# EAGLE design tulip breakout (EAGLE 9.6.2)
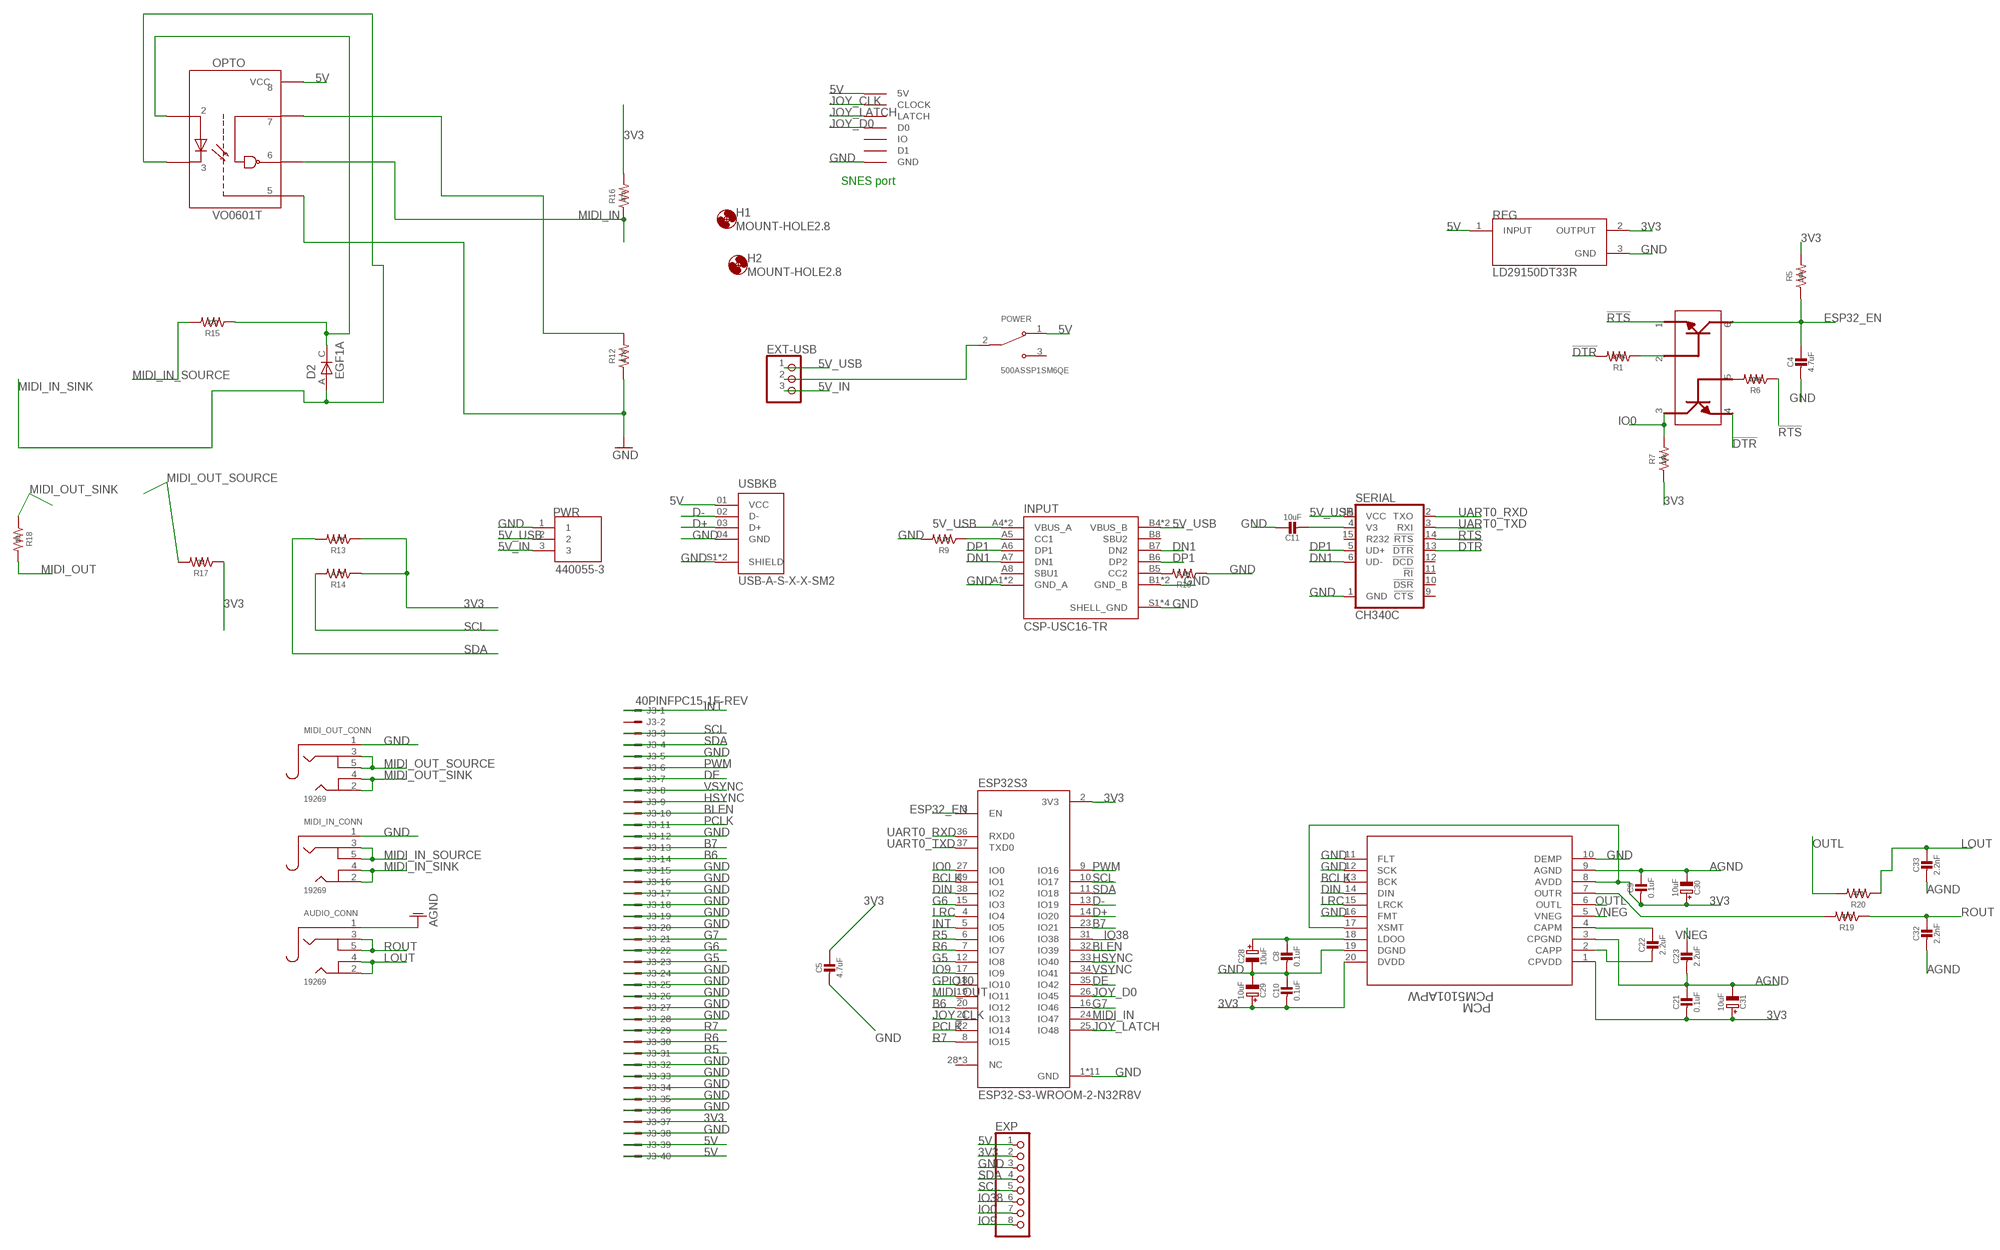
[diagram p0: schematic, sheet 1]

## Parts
AUDIO_CONN  19269  AUDIO_3.5MMJACK  [4UCONN_19269]
C4  4.7uF  CAP_CERAMIC0805-NOOUTLINE  [0805-NO]
C5  4.7uF  CAP_CERAMIC0805-NOOUTLINE  [0805-NO]
C8  0.1uF  CAP_CERAMIC0805-NOOUTLINE  [0805-NO]
C9  0.1uF  CAP_CERAMIC0805-NOOUTLINE  [0805-NO]
C10  0.1uF  CAP_CERAMIC0805-NOOUTLINE  [0805-NO]
C11  10uF  CAP_CERAMIC0805-NOOUTLINE  [0805-NO]
C21  0.1uF  CAP_CERAMIC0805-NOOUTLINE  [0805-NO]
C22  2.2uF  CAP_CERAMIC0805-NOOUTLINE  [0805-NO]
C23  2.2uF  CAP_CERAMIC0805-NOOUTLINE  [0805-NO]
C28  10uF  CAP_ELECTROLYTICPANASONIC_C  [PANASONIC_C]
C29  10uF  CAP_ELECTROLYTICPANASONIC_C  [PANASONIC_C]
C30  10uF  CAP_ELECTROLYTICPANASONIC_C  [PANASONIC_C]
C31  10uF  CAP_ELECTROLYTICPANASONIC_C  [PANASONIC_C]
C32  2.2nF  CAP_CERAMIC0805-NOOUTLINE  [0805-NO]
C33  2.2nF  CAP_CERAMIC0805-NOOUTLINE  [0805-NO]
D2  EGF1A  [DIOM449X264X300L114X135N]
ESP32S3  ESP32-S3-WROOM-2-N32R8V  [XCVR_ESP32-S3-WROOM-2-N32R8V]
EXP  PINHD-1X8BIG  [1X08-BIG]
EXT-USB  PINHD-1X3  [1X03]
H1  MOUNT-HOLE2.8  [2,8]
H2  MOUNT-HOLE2.8  [2,8]
INPUT  CSP-USC16-TR  [VALCON_CSP-USC16-TR]
J3  40PINFPC15-1F-REV  [XF2M-4015-1F-REVERSE]
MIDI_IN_CONN  19269  AUDIO_3.5MMJACK  [4UCONN_19269]
MIDI_OUT_CONN  19269  AUDIO_3.5MMJACK  [4UCONN_19269]
OPTO  VO0601T  [SOIC127P610X331-8N]
PCM  PCM5101APW  [PW20_TEX]
POWER  500ASSP1SM6QE  [SW_500ASSP1SM6QE]
PWR  440055-3  [TE_440055-3]
R1  100k  R-US_R0805  [R0805]
R5  10k  R-US_R0805  [R0805]
R6  100k  R-US_R0805  [R0805]
R7  10k  R-US_R0805  [R0805]
R9  5.1K  R-US_R0805  [R0805]
R10  5.1K  R-US_R0805  [R0805]
R12  4.7K  R-US_R0805  [R0805]
R13  4.7K  R-US_R0805  [R0805]
R14  4.7K  R-US_R0805  [R0805]
R15  220  R-US_R0805  [R0805]
R16  470  R-US_R0805  [R0805]
R17  33  R-US_R0805  [R0805]
R18  10  R-US_R0805  [R0805]
R19  470  R-US_R0805  [R0805]
R20  470  R-US_R0805  [R0805]
REG  LD29150DT33R  [DPAK456P972X240-3N]
RESET  MBT3904DW1T1G  [SOT236]
SERIAL  CH340C  [SO016]
SNES  SNESCONN  [SNESCONN]
USBKB  USB-A-S-X-X-SM2  [SAMTEC_USB-A-S-X-X-SM2]

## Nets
3V3: C5.1 C9.2 C10.2 C21.2 C29.+ C30.+ C31.+ ESP32S3.2(3V3) EXP.2 J3.37 PCM.1(CPVDD) PCM.8(AVDD) PCM.17(XSMT) PCM.20(DVDD) R5.2 R7.1 R13.1 R14.1 R16.2 R17.1 REG.2(OUTPUT)
5V: EXP.1 J3.39 J3.40 OPTO.8(VCC) POWER.1(NC) REG.1(INPUT) SNES.5V USBKB.01(VCC)
5V_IN: EXT-USB.3 PWR.3
5V_USB: EXT-USB.1 INPUT.A4(VBUS_A) INPUT.A9(VBUS_A) INPUT.B4(VBUS_B) INPUT.B9(VBUS_B) PWR.2 SERIAL.16(VCC)
!DTR: R1.2 RESET.4 SERIAL.13(!DTR)
!RTS: R6.1 RESET.1 SERIAL.14(!RTS)
AGND: AUDIO_CONN.1 C9.1 C21.1 C23.2 C30.- C31.- C32.2 C33.2 PCM.3(CPGND) PCM.9(AGND)
B6: ESP32S3.20(IO12) J3.14
B7: ESP32S3.23(IO21) J3.13
BCLK: ESP32S3.39(IO1) PCM.13(BCK)
BLEN: ESP32S3.32(IO39) J3.10
D+: ESP32S3.14(IO20) USBKB.03(D+)
D-: ESP32S3.13(IO19) USBKB.02(D-)
DE: ESP32S3.35(IO42) J3.7
DIN: ESP32S3.38(IO2) PCM.14(DIN)
DN1: INPUT.A7(DN1) INPUT.B7(DN2) SERIAL.6(UD-)
DP1: INPUT.A6(DP1) INPUT.B6(DP2) SERIAL.5(UD+)
ESP32_EN: C4.1 ESP32S3.3(EN) R5.1 RESET.6
EXT-USB: EXT-USB.2 POWER.2(COM)
G5: ESP32S3.12(IO8) J3.23
G6: ESP32S3.15(IO3) J3.22
G7: ESP32S3.16(IO46) J3.21
GND: C4.2 C5.2 C8.2 C10.1 C11.1 C28.- C29.- ESP32S3.1(GND) ESP32S3.40(GND) ESP32S3.41_1(GND) ESP32S3.41_2(GND) ESP32S3.41_3(GND) ESP32S3.41_4(GND) ESP32S3.41_5(GND) ESP32S3.41_6(GND) ESP32S3.41_7(GND) ESP32S3.41_8(GND) ESP32S3.41_9(GND) EXP.3 INPUT.A1(GND_A) INPUT.A12(GND_A) INPUT.B1(GND_B) INPUT.B12(GND_B) INPUT.S1(SHELL_GND) INPUT.S2(SHELL_GND) INPUT.S3(SHELL_GND) INPUT.S4(SHELL_GND) J3.5 J3.12 J3.15 J3.16 J3.17 J3.18 J3.19 J3.20 J3.24 J3.25 J3.26 J3.27 J3.28 J3.32 J3.33 J3.34 J3.35 J3.36 J3.38 MIDI_IN_CONN.1 MIDI_OUT_CONN.1 OPTO.5(GND) PCM.10(DEMP) PCM.11(FLT) PCM.12(SCK) PCM.16(FMT) PCM.19(DGND) PWR.1 R9.2 R10.1 R12.1 REG.3(GND) SERIAL.1(GND) SNES.GND USBKB.04(GND) USBKB.S1(SHIELD) USBKB.S2(SHIELD)
GPIO10: ESP32S3.18(IO10)
HSYNC: ESP32S3.33(IO40) J3.9
INT: ESP32S3.5(IO5) J3.1
IO0: ESP32S3.27(IO0) EXP.7 R7.2 RESET.3
IO9: ESP32S3.17(IO9) EXP.8
IO38: ESP32S3.31(IO38) EXP.6
JOY_CLK: ESP32S3.21(IO13) SNES.CLOCK
JOY_D0: ESP32S3.26(IO45) SNES.D0
JOY_LATCH: ESP32S3.25(IO48) SNES.LATCH
LOUT: AUDIO_CONN.2 AUDIO_CONN.4 C33.1 R20.1
LRC: ESP32S3.4(IO4) PCM.15(LRCK)
MIDI_IN: ESP32S3.24(IO47) OPTO.6(VO) R16.1
MIDI_IN_SINK: D2.A MIDI_IN_CONN.2 MIDI_IN_CONN.4 OPTO.3(C)
MIDI_IN_SOURCE: MIDI_IN_CONN.3 MIDI_IN_CONN.5 R15.2
MIDI_OUT: ESP32S3.19(IO11) R18.2
MIDI_OUT_SINK: MIDI_OUT_CONN.2 MIDI_OUT_CONN.4 R18.1
MIDI_OUT_SOURCE: MIDI_OUT_CONN.3 MIDI_OUT_CONN.5 R17.2
N$1: R1.1 RESET.2
N$2: R6.2 RESET.5
N$3: INPUT.B5(CC2) R10.2
N$7: C8.1 C28.+ PCM.18(LDOO)
N$8: PCM.7(OUTR) R19.2
N$16: C22.1 PCM.4(CAPM)
N$18: C22.2 PCM.2(CAPP)
N$30: D2.C OPTO.2(A) R15.1
N$32: OPTO.7(VE) R12.2
N$38: C11.2 SERIAL.4(V3)
N$42: INPUT.A5(CC1) R9.1
OUTL: PCM.6(OUTL) R20.2
PCLK: ESP32S3.22(IO14) J3.11
PWM: ESP32S3.9(IO16) J3.6
R5: ESP32S3.6(IO6) J3.31
R6: ESP32S3.7(IO7) J3.30
R7: ESP32S3.8(IO15) J3.29
ROUT: AUDIO_CONN.3 AUDIO_CONN.5 C32.1 R19.1
SCL: ESP32S3.10(IO17) EXP.5 J3.3 R14.2
SDA: ESP32S3.11(IO18) EXP.4 J3.4 R13.2
UART0_RXD: ESP32S3.36(RXD0) SERIAL.2(TXO)
UART0_TXD: ESP32S3.37(TXD0) SERIAL.3(RXI)
VNEG: C23.1 PCM.5(VNEG)
VSYNC: ESP32S3.34(IO41) J3.8
Unconnected: ESP32S3.28(NC) ESP32S3.29(NC) ESP32S3.30(NC) INPUT.A8(SBU1) INPUT.B8(SBU2) J3.2 POWER.3(NO) SERIAL.9(!CTS) SERIAL.10(!DSR) SERIAL.11(!RI) SERIAL.12(!DCD) SERIAL.15(R232) SNES.D1 SNES.IO

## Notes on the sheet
- SNES port

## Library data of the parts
AUDIO_CONN MIDI_IN_CONN MIDI_OUT_CONN = microbuilder:AUDIO_3.5MMJACK: 3.5MM Audio Jack These are normally connected as follows, from left-to right on the schematic symbol above: Tip: Left Audio Inner Ring: Right Audio Shell: Common/GND
C4 C5 C8-C11 C21-C23 C32 C33 = microbuilder:CAP_CERAMIC: Ceramic Capacitors
C28-C31 = microbuilder:CAP_ELECTROLYTIC: Electrolytic Capacitors
D2 = EGF1A:EGF1A: EGF1A Series 1 A 100 V 50 ns Surface Mount Fast Recovery Rectifier - DO-214AC Check availability; AVAILABILITY: In Stock; DESCRIPTION: Diode Standard 50 V 1A Surface Mount DO-214AC (SMA); MF: ON Semiconductor; MP: EGF1A; PACKAGE: SMA-2 ON Semiconductor; PRICE: None; PURCHASE-URL: https://pricing.snapeda.com/search/part/EGF1A/?ref=eda
ESP32S3 = ESP32-S3-WROOM-2-N32R8V:ESP32-S3-WROOM-2-N32R8V: Check availability; AVAILABILITY: In Stock; DESCRIPTION: Bluetooth, WiFi 802.11b/g/n, Bluetooth v5.0 Transceiver Module 2.4GHz PCB Trace Surface Mount; MF: Espressif Systems; MP: ESP32-S3-WROOM-2-N32R8V; PACKAGE: Package; PRICE: None; PURCHASE-URL: https://pricing.snapeda.com/search/part/ESP32-S3-WROOM-2-N32R8V/?ref=eda
EXP = adafruit:PINHD-1X8: PIN HEADER
EXT-USB = adafruit:PINHD-1X3: PIN HEADER
H1 H2 = holes:MOUNT-HOLE: MOUNTING HOLE with drill center marker
INPUT = CSP-USC16-TR:CSP-USC16-TR: CSP-USC16-TR Valcon USB Type C Surface Mount PCB Socket Check availability; AVAILABILITY: In Stock; DESCRIPTION: CSP-USC16-TR Valcon USB Type C Surface Mount PCB Socket; MF: Valcon; MP: CSP-USC16-TR; PACKAGE: None; PRICE: None; PURCHASE-URL: https://pricing.snapeda.com/search/part/CSP-USC16-TR/?ref=eda
J3 = adafruit:40PINFPC: OMRON FPC Connector Source : http://www.omron.com/ecb/products/pdf/fpc.pdf XF2M-4015-rev is good for connecting up 'PSP' SHARP LQ043 LCDs
OPTO = VO0601T:VO0601T: High Speed Optocoupler, 10 MBd, SOIC-8 Package; DESCRIPTION: Logic Output Optoisolator 10MBd Open Drain 4000Vrms 1 Channel 5kV/µs CMTI 8-SOIC; DIGI-KEY_PART_NUMBER: 751-1377-2-ND; MF: Vishay Semiconductors; MP: VO0601T; PACKAGE: None; PURCHASE-URL: https://pricing.snapeda.com/search/part/VO0601T/?ref=eda
PCM = pcm5101apw:PCM5101APW; COPYRIGHT: Copyright (C) 2022 Ultra Librarian. All rights reserved.; DIGI-KEY_PART_NUMBER_1: PCM5101APW-ND; MANUFACTURER_PART_NUMBER: PCM5101APW; MFR_NAME: Texas Instruments
POWER = 500ASSP1SM6QE:500ASSP1SM6QE; DESCRIPTION: Slide Switch SPDT Surface Mount, Right Angle; DIGI-KEY_PART_NUMBER: EG5810TR-ND; MF: E-Switch; MP: 500ASSP1SM6QE; PACKAGE: None; PURCHASE-URL: https://pricing.snapeda.com/search/part/500ASSP1SM6QE/?ref=eda
PWR = 440055-3:440055-3; COMMENT: 440055-3; DESCRIPTION: Connector Header Through Hole, Right Angle 3 position 0.079 (2.00mm); DIGI-KEY_PART_NUMBER: A100044-ND; EU_ROHS_COMPLIANCE: Compliant; MF: TE Connectivity; MP: 440055-3; PACKAGE: None; PURCHASE-URL: https://pricing.snapeda.com/search/part/440055-3/?ref=eda
R1 R5-R7 R9 R10 R12-R20 = adafruit:R-US_: RESISTOR, American symbol
REG = LD29150DT33R:LD29150DT33R: LD29150 Series 1.5 A 3.3 V Fixed Output SMT LDO Voltage Regulator - TO-252; DESCRIPTION: Linear Voltage Regulator IC Positive Fixed 1 Output 1.5A DPAK; DIGI-KEY_PART_NUMBER: 497-1496-2-ND; MF: STMicroelectronics; MP: LD29150DT33R; PACKAGE: TO-252 STMicroelectronics; PURCHASE-URL: https://pricing.snapeda.com/search/part/LD29150DT33R/?ref=eda
RESET = MBT3904DW1T1G:MBT3904DW1T1G: Check availability; AVAILABILITY: In Stock; DESCRIPTION: Bipolar (BJT) Transistor Array 2 NPN (Dual) 40V 200mA 300MHz 150mW Surface Mount SC-88/SC70-6/SOT-363; MF: ON Semiconductor; MP: MBT3904DW1T1G; PACKAGE: SC-88-6 ON Semiconductor; PRICE: None; PURCHASE-URL: https://pricing.snapeda.com/search/part/MBT3904DW1T1G/?ref=eda
SERIAL = SparkFun-IC-Comms:CH340C; PROD_ID: IC-14038
SNES = gamepad-conn:SNESCONN
USBKB = USB-A-S-X-X-SM2:USB-A-S-X-X-SM2: USB-A (USB TYPE-A) USB 2.0 Receptacle Connector 4 Position Surface Mount, Right Angle; Through Hole Check availability; AVAILABILITY: In Stock; DESCRIPTION: USB-A (USB TYPE-A) USB 2.0 Receptacle Connector 4 Position Surface Mount, Right Angle; MF: Samtec; MP: USB-A-S-F-W-SM2-TR; PACKAGE: None; PRICE: None; PURCHASE-URL: https://pricing.snapeda.com/search/part/USB-A-S-F-W-SM2-TR/?ref=eda

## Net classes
1 power: width 0.178 mm

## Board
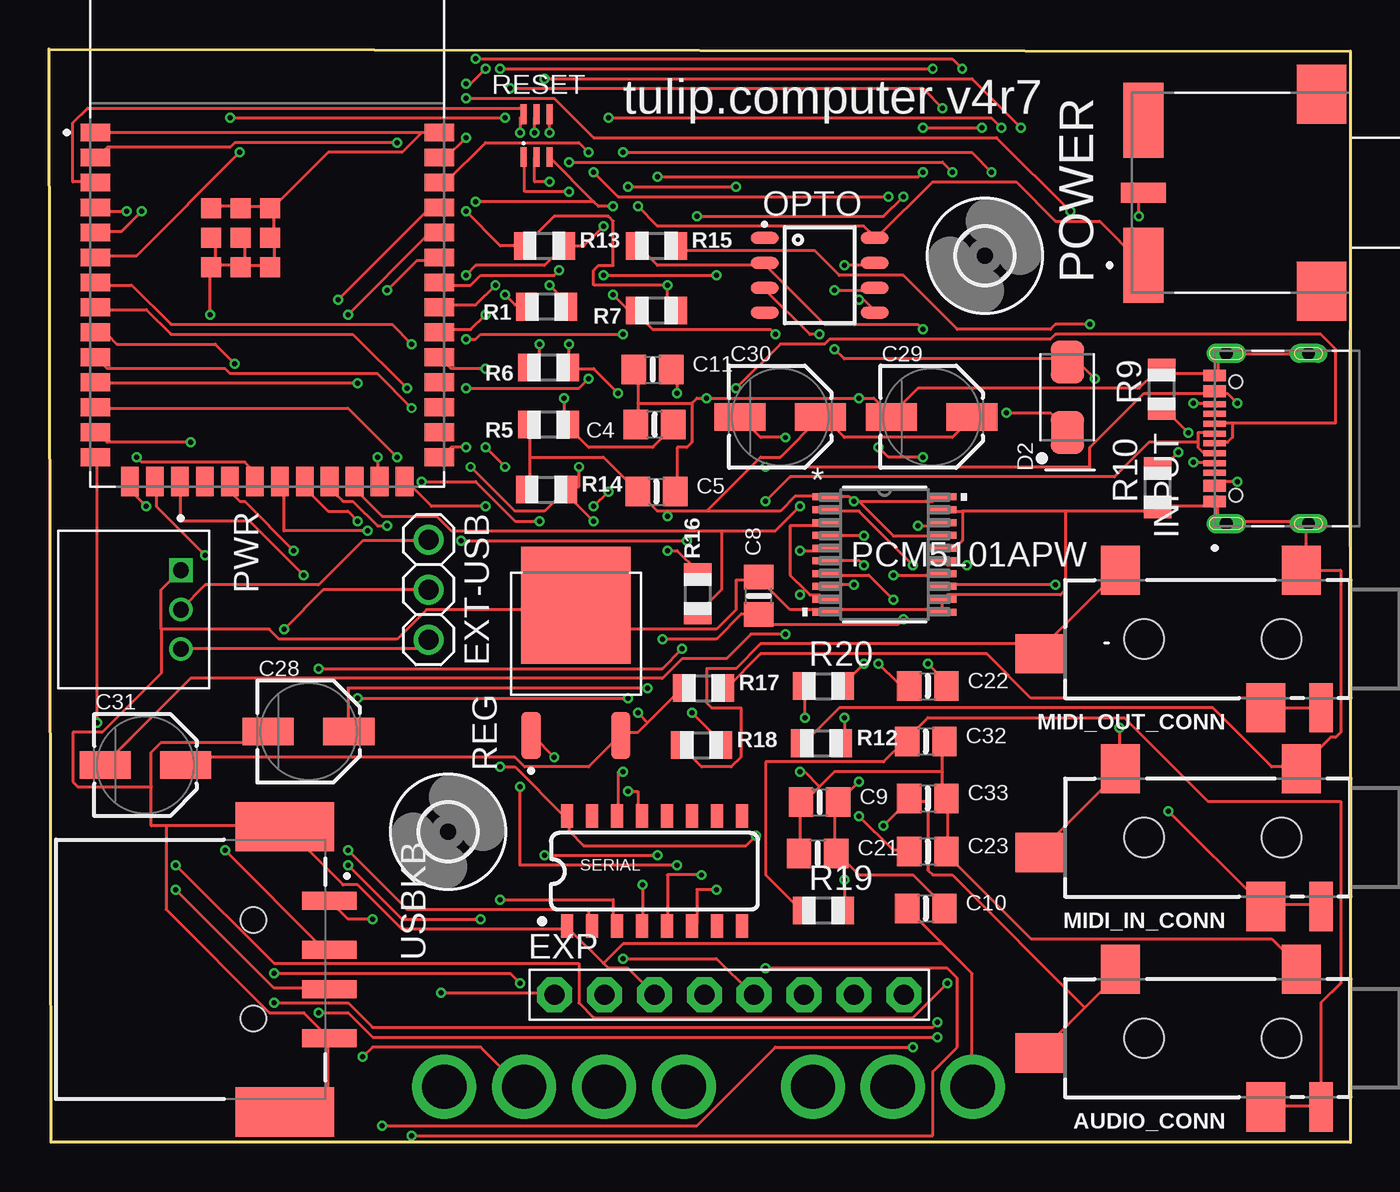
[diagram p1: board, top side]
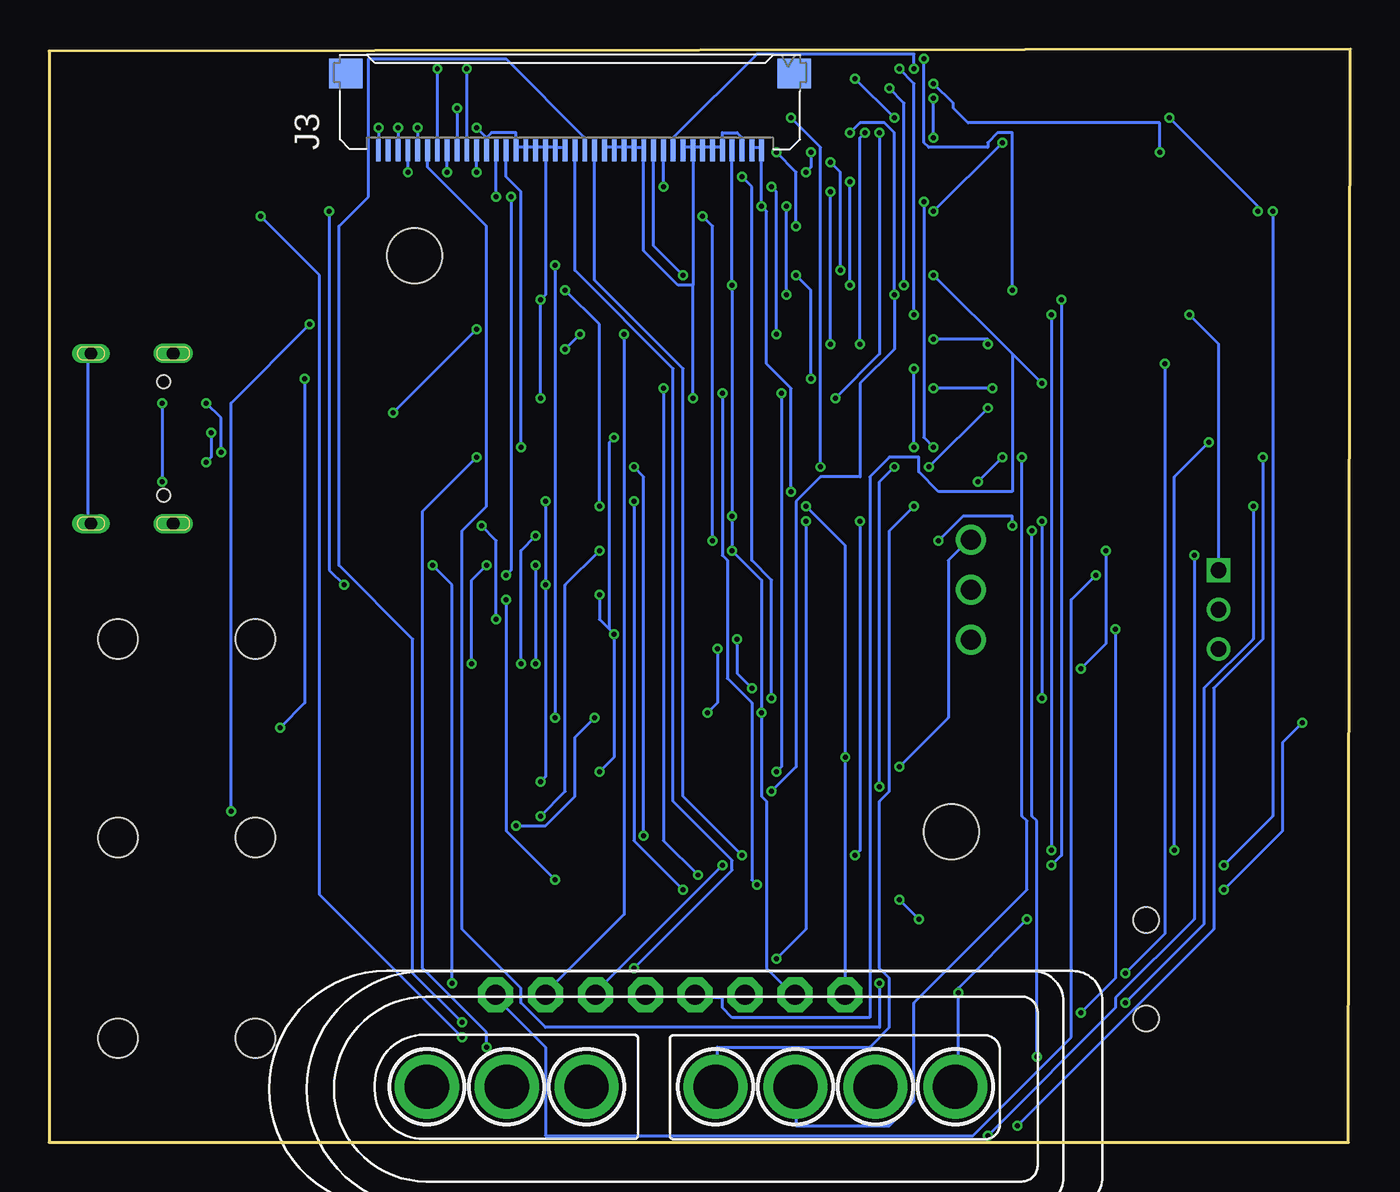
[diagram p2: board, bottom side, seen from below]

Size 66.2 x 55.6 mm. Coordinates in mm from the lower left corner, seen from the top.
Outline: 0.1,0 0,55.6 66.2,55.5 66.2,0 0.1,0
Copper layers (1*16): Top 0.035559375mm / dielectric 1.6mm / Bottom 0.035559375mm
Design rules "oshpark-2layer *": minimum track width 6mil, minimum drill 10mil, track to track 6mil, track to pad 6mil, pad to pad 6mil, via to via 6mil, smd to smd 6mil, copper to edge 0mil, drill to drill 6mil, minimum pad ring 5mil, minimum via ring 5mil, stop-mask expansion 2.5mil, vias tented up to drill 0mil, thermal gap 10mil

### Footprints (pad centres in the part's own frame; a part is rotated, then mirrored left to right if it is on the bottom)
4UCONN_19269 = smd 2 x 2.5: 1 2.5,-3.5; 2 11.7,-3.5; 3 4.3,3.5 | smd 2.5 x 2: 4 15.8,0.75 | smd 1.2 x 2.5: 5 1.5,3.5 | hole 2: 3.5,0; 10.5,0
0805-NO = smd 1.24 x 1.5: 1 -0.95,0; 2 0.95,0
PANASONIC_C = smd 2.6 x 1.4: + 2.05,0; - -2.05,0
DIOM449X264X300L114X135N = smd 2.17 x 1.69: A 1.795,0; C -1.795,0
XCVR_ESP32-S3-WROOM-2-N32R8V = smd 1.5 x 0.9: 1 -8.75,5.26; 2 -8.75,3.99; 3 -8.75,2.72; 4 -8.75,1.45; 5 -8.75,0.18; 6 -8.75,-1.09; 7 -8.75,-2.36; 8 -8.75,-3.63; 9 -8.75,-4.9; 10 -8.75,-6.17; 11 -8.75,-7.44; 12 -8.75,-8.71; 13 -8.75,-9.98; 14 -8.75,-11.25; 27 8.75,-11.25; 28 8.75,-9.98; 29 8.75,-8.71; 30 8.75,-7.44; 31 8.75,-6.17; 32 8.75,-4.9; 33 8.75,-3.63; 34 8.75,-2.36; 35 8.75,-1.09; 36 8.75,0.18; 37 8.75,1.45; 38 8.75,2.72; 39 8.75,3.99; 40 8.75,5.26 | smd 0.9 x 1.5: 15 -6.985,-12.5; 16 -5.715,-12.5; 17 -4.445,-12.5; 18 -3.175,-12.5; 19 -1.905,-12.5; 20 -0.635,-12.5; 21 0.635,-12.5; 22 1.905,-12.5; 23 3.175,-12.5; 24 4.445,-12.5; 25 5.715,-12.5; 26 6.985,-12.5 | smd 1 x 1: 41_1 -1.36,-0.09; 41_2 -2.86,-0.09; 41_3 0.14,-0.09; 41_4 -2.86,-1.59; 41_5 -1.36,-1.59; 41_6 0.14,-1.59; 41_7 -2.86,1.41; 41_8 -1.36,1.41; 41_9 0.14,1.41
1X08-BIG = drill 1.016 pad 1.778 octagon: 1 -8.89,0; 2 -6.35,0; 3 -3.81,0; 4 -1.27,0; 5 1.27,0; 6 3.81,0; 7 6.35,0; 8 8.89,0
1X03 = drill 1.016: 1 -2.54,0; 2 0,0; 3 2.54,0
2,8 = hole 2.8: 0,0
VALCON_CSP-USC16-TR = smd 0.3 x 1.14: A1 -3.35,0; A4 -2.55,0; A5 -1.25,0; A6 -0.25,0; A7 0.25,0; A8 1.25,0; A9 2.55,0; A12 3.35,0; B1 3.05,0; B4 2.25,0; B5 1.75,0; B6 0.75,0; B7 -0.75,0; B8 -1.75,0; B9 -2.25,0; B12 -3.05,0 | drill 0.65 pad 1 long: S1 -4.325,-0.59; S2 4.325,-0.59 | drill 0.65 pad 0.9 long: S3 -4.325,-4.77; S4 4.325,-4.77 | hole 0.65: -2.89,-1.07; 2.89,-1.07
XF2M-4015-1F-REVERSE = smd 1.1 x 0.25: 1 -2.54,9.75; 2 -2.54,9.25; 3 -2.54,8.75; 4 -2.54,8.25; 5 -2.54,7.75; 6 -2.54,7.25; 7 -2.54,6.75; 8 -2.54,6.25; 9 -2.54,5.75; 10 -2.54,5.25; 11 -2.54,4.75; 12 -2.54,4.25; 13 -2.54,3.75; 14 -2.54,3.25; 15 -2.54,2.75; 16 -2.54,2.25; 17 -2.54,1.75; 18 -2.54,1.25; 19 -2.54,0.75; 20 -2.54,0.25; 21 -2.54,-0.25; 22 -2.54,-0.75; 23 -2.54,-1.25; 24 -2.54,-1.75; 25 -2.54,-2.25; 26 -2.54,-2.75; 27 -2.54,-3.25; 28 -2.54,-3.75; 29 -2.54,-4.25; 30 -2.54,-4.75; 31 -2.54,-5.25; 32 -2.54,-5.75; 33 -2.54,-6.25; 34 -2.54,-6.75; 35 -2.54,-7.25; 36 -2.54,-7.75; 37 -2.54,-8.25; 38 -2.54,-8.75; 39 -2.54,-9.25; 40 -2.54,-9.75 | smd 1.5 x 1.7: M1 1.36,11.4; M2 1.36,-11.4
SOIC127P610X331-8N = smd 1.4 x 0.6: 1 -2.8,1.905; 2 -2.8,0.635; 3 -2.8,-0.635; 4 -2.8,-1.905; 5 2.8,-1.905; 6 2.8,-0.635; 7 2.8,0.635; 8 2.8,1.905
PW20_TEX = smd 1.473 x 0.356: 1 -2.921,2.925; 2 -2.921,2.275; 3 -2.921,1.625; 4 -2.921,0.975; 5 -2.921,0.325; 6 -2.921,-0.325; 7 -2.921,-0.975; 8 -2.921,-1.625; 9 -2.921,-2.275; 10 -2.921,-2.925; 11 2.921,-2.925; 12 2.921,-2.275; 13 2.921,-1.625; 14 2.921,-0.975; 15 2.921,-0.325; 16 2.921,0.325; 17 2.921,0.975; 18 2.921,1.625; 19 2.921,2.275; 20 2.921,2.925
SW_500ASSP1SM6QE = smd 3.81 x 2.03: 1 -3.685,4.535; 3 3.685,4.535 | smd 1.02 x 2.29: 2 0,4.535 | smd 3 x 2.5: S1 -5,-4.535; S2 5,-4.535
TE_440055-3 = drill 0.8 pad 1.15 square: 1 0,0 | drill 0.8 pad 1.15: 2 2.007,0; 3 4.013,0
R0805 = smd 1.1 x 1.4: 1 -1,0; 2 1,0
DPAK456P972X240-3N = smd 2.4 x 0.98: 1 -4.2,2.28; 2 -4.2,-2.28 | smd 5.96 x 5.57: 3 2.42,0
SOT236 = smd 0.3 x 1: 1 -0.66,-1.09; 2 0,-1.09; 3 0.66,-1.09; 4 0.66,1.09; 5 0,1.09; 6 -0.66,1.09
SO016 = smd 0.6 x 1.2: 1 -4.445,-2.8; 2 -3.175,-2.8; 3 -1.905,-2.8; 4 -0.635,-2.8; 5 0.635,-2.8; 6 1.905,-2.8; 7 3.175,-2.8; 8 4.445,-2.8; 9 4.445,2.8; 10 3.175,2.8; 11 1.905,2.8; 12 0.635,2.8; 13 -0.635,2.8; 14 -1.905,2.8; 15 -3.175,2.8; 16 -4.445,2.8
SNESCONN = drill 2.25 pad 3.25: 5V 0,4.064; CLOCK 4.064,4.064; D0 12.192,4.064; D1 18.756,4.064; GND 26.884,4.064; IO 22.82,4.064; LATCH 8.128,4.064
SAMTEC_USB-A-S-X-X-SM2 = smd 0.9 x 2.8: 01 -3.5,3.85; 02 -1,3.85; 03 1,3.85; 04 3.5,3.85 | smd 2.5 x 5: S1 -7.25,1.6; S2 7.25,1.6 | hole 1.3: -2.5,0; 2.5,0

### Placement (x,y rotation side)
AUDIO_CONN  66.2,5.3 180 top
C4  30.8,36.5 180 top
C5  30.9,33.1 0 top
C8  36.1,27.8 90 top
C9  39.2,17.3 0 top
C10  44.6,11.9 0 top
C11  30.7,39.3 0 top
C21  39.1,14.7 0 top
C22  44.7,23.2 0 top
C23  44.7,14.8 0 top
C28  13.2,20.9 0 top
C29  44.9,36.9 0 top
C30  37.2,36.9 0 top
C31  4.9,19.2 0 top
C32  44.6,20.4 0 top
C33  44.7,17.5 0 top
D2  51.8,37.9 90 top
ESP32S3  11.1,46.1 0 top
EXP  34.6,7.5 0 top
EXT-USB  19.3,28.1 270 top
H1  20.3,15.8 0 top
H2  47.6,45.1 0 top
INPUT  59.3,35.8 90 top
J3  39.7,53 90 bottom
MIDI_IN_CONN  66.2,15.5 180 top
MIDI_OUT_CONN  66.2,25.6 180 top
OPTO  39.2,44.1 0 top
PCM  42.5,29.9 0 top
POWER  60.2,48.3 90 top
PWR  6.7,29.1 270 top
R1  25.3,42.5 180 top
R5  25.4,36.5 180 top
R6  25.4,39.4 180 top
R7  30.9,42.3 180 top
R9  56.6,38.3 90 top
R10  56.4,33.3 90 top
R12  39.3,20.3 0 top
R13  25.2,45.6 0 top
R14  25.3,33.2 0 top
R15  30.9,45.6 0 top
R16  33,27.9 90 top
R17  33.3,23.1 0 top
R18  33.2,20.2 0 top
R19  39.4,11.8 0 top
R20  39.4,23.2 0 top
REG  26.8,24.9 90 top
RESET  24.8,51.2 0 top
SERIAL  30.8,13.8 0 top
SNES  20.1,6.9 180 bottom
USBKB  10.4,8.8 270 top

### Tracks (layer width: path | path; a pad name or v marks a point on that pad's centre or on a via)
3V3  (via drill 0.25)
  Top 0.152: C29.+ 46.95,36.85 45.95,35.85 40.45,35.85 39.45,36.85 C30.+ 37.2,34.85 36.2,34.85 33.45,32.1 | C10.2 45.45,12.1 43.95,13.6 41.2,13.6 40.2,14.6 C21.2 39.95,14.85 39.95,17.1 C9.2 v41.2,18.35 | 24.45,34.85 24.45,36.35 R5.2 | 24.45,34.85 24.45,33.35 R14.1 | 24.45,34.85 28.2,34.85 C5.1 30.95,32.1 31.45,32.1 | v40.95,28.35 39.7,28.35 PCM.8 | 41.2,32.6 42.95,30.85 45.2,30.85 PCM.17 | 41.2,32.6 44.95,32.6 45.2,32.85 PCM.20 | 41.2,32.6 v40.95,32.6 40.7,32.85 39.7,32.85 PCM.1 39.45,32.85 37.95,32.85 37.2,32.1 33.45,32.1 | 33.45,32.1 31.45,32.1 | 30.45,21.35 29.95,20.85 29.2,20.85 REG.2 28.95,20.6 27.45,19.1 24.2,19.1 23.7,19.6 7.2,19.6 6.95,19.35 C31.+ | 30.45,21.35 32.2,23.1 R17.1 | R7.1 31.7,42.35 31.45,42.35 v31.45,43.6 27.7,43.6 27.7,44.35 27.95,44.6 28.7,44.6 28.7,46.85 28.45,47.1 25.7,47.1 R13.1 22.95,45.6 v21.2,47.35 | v31.45,30.1 31.95,30.1 32.95,29.1 R16.2 | v17.7,50.85 9.45,50.85 9.2,50.6 2.95,50.6 2.45,50.1 ESP32S3.2 | v29.95,21.85 30.45,21.35 | v31.45,31.85 31.45,32.1
  Bottom 0.152: v40.95,32.6 v40.95,28.35 40.95,18.6 v41.2,18.35 | J3.37 v31.45,43.6 v31.45,31.85 v31.45,30.1 29.95,28.6 v29.95,21.85 29.95,17.6 29.7,17.35 29.7,8.85 28.45,7.6 EXP.2 | v21.2,47.35 v17.7,50.85
5V  (via drill 0.25)
  Top 0.152: v29.95,47.6 30.95,46.6 41.45,46.6 41.95,46.1 OPTO.8 42.2,46.1 44.95,48.85 49.2,48.85 51.2,46.85 53.45,46.85 55.45,44.85 POWER.1 | v25.7,19.6 24.7,20.6 REG.1 | USBKB.01 15.2,11.35 v16.45,11.35 | v19.95,7.6 25.7,7.6 EXP.1 | v27.7,32.35 v28.45,33.1
  Bottom 0.152: J3.39 30.45,50.6 29.95,50.6 J3.40 v29.95,47.6 29.7,47.35 29.7,39.6 28.45,38.35 v28.45,33.1 | EXP.1 25.7,7.6 v25.7,19.6 25.7,30.35 v27.7,32.35 | v16.45,11.35 19.95,7.85 v19.95,7.6 19.95,2.85 SNES.5V
5V_IN
  Top 0.152: PWR.3 18.95,25.1 19.2,25.35 EXT-USB.3
5V_USB  (via drill 0.25)
  Top 0.152: 59.45,33.6 59.45,33.35 INPUT.A4 | 59.45,38.1 59.45,38.35 INPUT.A9 | v60.45,33.6 59.45,33.6 | v60.45,37.6 59.95,38.1 59.45,38.1 | 59.45,33.6 INPUT.B9 | 59.45,38.1 INPUT.B4 59.2,38.1 55.7,38.1 52.95,35.35 52.95,34.35 v36.45,34.35 | v22.95,19.1 23.7,19.1 26.2,16.6 SERIAL.16 26.45,16.6 26.45,15.85 27.2,15.1 35.45,15.1 v35.95,15.6 | PWR.2 7.95,28.35 13.7,28.35 15.95,30.6 19.2,30.6 EXT-USB.1
  Bottom 0.152: v60.45,37.6 v60.45,33.6 | v22.95,19.1 20.45,21.6 20.45,29.6 19.45,30.6 EXT-USB.1 | v36.45,34.35 35.95,33.85 v35.95,15.6
!DTR  (via drill 0.25)
  Top 0.152: v25.45,51.35 25.45,52.1 RESET.4 | v23.2,43.1 23.7,42.6 24.2,42.6 R1.2 | v29.45,17.85 29.95,17.85 29.95,16.6 SERIAL.13
  Bottom 0.152: v25.45,51.35 24.95,51.85 23.7,51.85 23.2,51.35 v23.2,43.1 23.2,40.35 24.95,38.6 24.95,33.85 26.95,33.85 28.2,32.6 28.2,19.1 v29.45,17.85
!RTS  (via drill 0.25)
  Top 0.152: v26.45,48.35 24.2,48.35 24.2,50.1 RESET.1 | v26.45,40.6 26.45,39.6 R6.1 26.45,39.35 27.7,39.35 v28.95,38.1 | v29.2,18.85 28.95,18.85 28.95,16.6 SERIAL.14
  Bottom 0.152: v26.45,40.6 v26.45,48.35 | v29.2,18.85 28.95,19.1 v28.95,38.1
AGND  (via drill 0.25)
  Top 0.152: C21.1 38.2,14.85 38.2,17.1 C9.1 38.45,17.35 39.2,18.1 | 45.45,18.85 45.45,17.6 C33.2 45.7,17.35 45.7,14.85 C23.2 45.7,14.6 49.95,10.35 62.2,10.35 63.7,8.85 AUDIO_CONN.1 | 45.45,18.85 45.45,20.35 C32.2 | 39.2,18.1 39.95,18.85 45.45,18.85 | 38.45,28.1 37.7,28.85 37.7,31.35 39.45,31.35 PCM.3 | 38.45,28.1 38.7,27.85 39.2,27.85 39.45,27.6 PCM.9 | v37.45,25.85 35.7,25.85 34.45,24.6 32.2,24.6 31.2,23.6 7.2,23.6 2.95,19.35 C31.- | 38.45,28.1 v38.2,27.85 | C30.- 36.2,35.85 v37.45,35.85 | 39.2,18.1 38.45,18.85 v38.2,18.85
  Bottom 0.152: 37.7,26.1 38.2,26.6 v38.2,27.85 | 37.7,26.1 v37.45,25.85 37.45,19.6 v38.2,18.85 | v37.45,35.85 37.7,35.6 37.7,26.1
B6  (via drill 0.25)
  Top 0.152: v42.2,35.35 42.7,34.85 v44.45,34.85 | v43.95,4.85 36.95,4.85 32.95,0.85 v16.95,0.85 | v4.45,34.85 4.7,34.6 9.95,34.6 10.45,34.1 10.45,33.6 ESP32S3.20
  Bottom 0.152: J3.14 42.95,49.1 42.2,48.35 v42.2,35.35 | v44.45,34.85 47.2,32.1 47.2,8.85 43.95,5.6 v43.95,4.85 | v16.95,0.85 6.95,10.85 6.95,23.1 4.45,25.6 v4.45,34.85
B7  (via drill 0.25)
  Top 0.152: v43.45,48.1 42.45,47.1 v32.95,47.1 | v20.95,30.6 v32.45,30.6 | v17.2,31.35 16.7,31.35 15.45,32.6 14.95,32.6 14.45,33.1 14.45,33.6 ESP32S3.23
  Bottom 0.152: v43.45,48.1 J3.13 | v32.95,47.1 32.45,46.6 v32.45,30.6 | v20.95,30.6 19.7,31.85 17.2,31.85 v17.2,31.35
BCLK  (via drill 0.25)
  Top 0.152: v51.2,28.35 45.45,28.35 PCM.13 | v51.95,47.35 48.2,51.1 27.7,51.1 25.7,53.1 v21.2,53.1 | v21.2,51.1 20.2,50.1 19.95,50.1 ESP32S3.39
  Bottom 0.152: v51.2,28.35 51.95,29.1 v51.95,47.35 | v21.2,51.1 v21.2,53.1
BLEN  (via drill 0.25)
  Top 0.152: v22.95,54.6 v44.95,54.6 | v22.2,42.1 21.45,41.35 19.95,41.35 ESP32S3.32
  Bottom 0.152: v44.95,54.6 J3.10 | v22.95,54.6 22.2,53.85 v22.2,42.1
D+  (via drill 0.25)
  Top 0.152: v2.45,21.35 2.45,34.85 ESP32S3.14 | v6.45,12.85 11.45,7.85 14.2,7.85 USBKB.03
  Bottom 0.152: v2.45,21.35 3.45,20.35 3.45,15.85 v6.45,12.85
D-  (via drill 0.25)
  Top 0.152: v7.2,35.6 2.95,35.6 2.45,36.1 ESP32S3.13 | v8.95,14.85 13.95,9.85 14.2,9.85 USBKB.02
  Bottom 0.152: v7.2,35.6 8.95,33.85 v8.95,14.85
DE  (via drill 0.25)
  Top 0.152: v46.45,54.6 45.95,55.1 v21.7,55.1 | v17.2,43.35 18.7,44.85 19.7,44.85 ESP32S3.35
  Bottom 0.152: v46.45,54.6 J3.7 | v21.7,55.1 21.7,50.85 21.45,50.6 18.45,50.6 18.45,50.85 17.95,51.35 17.2,51.35 v17.2,43.35
DIN  (via drill 0.25)
  Top 0.152: v42.95,28.85 45.2,28.85 PCM.14 | v42.7,48.1 28.95,48.1 v27.7,49.35 | v27.45,50.35 26.95,50.85 22.2,50.85 20.2,48.85 19.95,48.85 ESP32S3.38
  Bottom 0.152: v42.95,28.85 42.7,29.1 v42.7,48.1 | v27.7,49.35 27.45,49.6 v27.45,50.35
DN1  (via drill 0.25)
  Top 0.152: 58.45,35.6 58.45,36.1 59.2,36.1 INPUT.A7 | 58.45,35.6 58.45,35.35 58.7,35.1 59.2,35.1 INPUT.B7 | v33.95,12.85 32.95,12.85 32.95,11.1 SERIAL.6 | v36.45,32.6 37.7,33.85 54.2,33.85 55.95,35.6 58.45,35.6
  Bottom 0.152: v33.95,12.85 36.45,15.35 v36.45,32.6
DP1  (via drill 0.25)
  Top 0.152: 60.2,36.6 60.2,35.85 59.95,35.6 59.45,35.6 INPUT.A6 | 60.2,36.6 59.45,36.6 INPUT.B6 | v33.2,13.6 31.45,13.6 31.45,11.1 SERIAL.5 | v34.95,38.35 37.2,40.6 39.45,40.6 39.7,40.85 50.95,40.85 51.2,41.1 64.7,41.1 65.45,40.35 65.45,36.6 60.2,36.6
  Bottom 0.152: v33.2,13.6 34.95,15.35 v34.95,38.35
ESP32_EN  (via drill 0.25)
  Top 0.152: C4.1 31.7,36.35 30.7,35.35 27.45,35.35 26.45,36.35 R5.1 26.2,36.6 v26.2,37.85 | ESP32S3.3 2.2,48.85 1.2,48.85 1.2,51.85 1.95,52.6 23.95,52.6 24.2,52.35 RESET.6 24.2,52.1 23.95,52.1 v23.95,51.35
  Bottom 0.152: v26.2,37.85 23.95,40.1 v23.95,51.35
EXT-USB  (via drill 0.25)
  Top 0.152: v55.45,47.1 55.45,48.1 POWER.2 | v45.2,5.35 16.45,5.35 15.2,6.6 v13.7,6.6 | v11.95,26.1 13.95,28.1 EXT-USB.2
  Bottom 0.152: v55.45,47.1 52.45,44.1 52.45,12.6 v45.2,5.35 | v13.7,6.6 11.95,8.35 v11.95,26.1
G5  (via drill 0.25)
  Top 0.152: v25.2,14.6 v30.95,14.6 | v24.95,31.6 23.7,31.6 21.7,33.6 v18.95,33.6 | v17.7,34.85 15.2,37.35 2.45,37.35 ESP32S3.12
  Bottom 0.152: J3.23 38.45,43.85 33.95,39.35 33.95,17.6 v30.95,14.6 | v25.2,14.6 24.95,14.85 v24.95,31.6 | v17.7,34.85 v18.95,33.6
G6  (via drill 0.25)
  Top 0.152: v45.2,6.1 44.95,5.85 16.45,5.85 15.2,7.1 v11.45,7.1 | v4.95,32.35 4.2,33.1 4.2,33.6 ESP32S3.15
  Bottom 0.152: J3.22 38.95,51.1 42.95,55.1 49.95,55.1 49.95,48.1 51.45,46.6 51.45,29.35 47.7,25.6 47.7,8.6 v45.2,6.1 | v11.45,7.1 7.45,11.1 7.45,23.1 4.95,25.6 v4.95,32.35
G7  (via drill 0.25)
  Top 0.152: v36.45,8.85 45.7,8.85 46.2,8.35 46.2,4.85 44.95,3.6 44.95,0.35 v18.45,0.35 | v7.95,29.85 5.45,32.35 5.45,33.6 ESP32S3.16
  Bottom 0.152: J3.21 39.45,44.35 34.45,39.35 34.45,17.35 31.45,14.35 31.45,13.85 v36.45,8.85 | v18.45,0.35 11.95,6.85 11.95,7.35 7.95,11.35 v7.95,29.85
GND  (via drill 0.25)
  Top 0.152: USBKB.S2 12.2,1.6 14.2,1.6 14.2,5.1 USBKB.04 12.95,6.6 11.2,6.6 5.95,11.85 5.95,16.1 | 5.2,18.1 5.2,16.1 5.95,16.1 | 5.2,18.1 5.2,19.85 5.7,20.35 10.45,20.35 10.95,20.85 C28.- | 5.95,16.1 11.95,16.1 USBKB.S1 14.95,13.1 15.7,13.1 17.95,10.85 26.2,10.85 SERIAL.1 26.45,10.85 28.2,9.1 | 28.2,9.1 28.45,8.85 29.45,8.85 30.7,7.6 EXP.3 | 45.45,10.1 46.95,8.6 46.95,2.85 SNES.GND | 45.45,10.1 C10.1 | 28.2,9.1 29.2,10.1 45.45,10.1 | ESP32S3.41_7 8.45,47.6 9.7,47.6 ESP32S3.41_8 9.95,47.6 11.2,47.6 ESP32S3.41_9 | 8.45,44.6 8.45,45.85 ESP32S3.41_2 | 9.95,44.6 9.95,45.85 ESP32S3.41_1 | 8.45,44.6 9.7,44.6 ESP32S3.41_5 9.95,44.6 | 8.45,44.6 ESP32S3.41_4 8.2,44.35 v8.2,42.1 | 9.95,44.6 11.2,44.6 ESP32S3.41_6 11.45,44.6 11.45,45.85 ESP32S3.41_3 11.45,46.1 11.45,47.35 ESP32S3.41_9 | 18.95,51.35 19.7,51.35 ESP32S3.40 | 18.95,51.35 2.45,51.35 ESP32S3.1 | 18.95,51.35 17.95,50.35 14.2,50.35 11.45,47.6 ESP32S3.41_9 | PWR.1 5.7,28.1 5.7,26.1 | 5.7,26.1 11.2,26.1 11.7,25.6 17.7,25.6 19.2,27.1 26.7,27.1 REG.3 26.95,27.1 27.95,26.1 33.95,26.1 34.95,27.1 34.95,28.6 35.95,28.6 C8.2 36.2,28.6 37.7,27.1 39.45,27.1 PCM.10 39.7,27.1 45.2,27.1 PCM.11 45.45,27.1 45.45,27.6 | v44.45,51.6 v47.45,51.6 | v41.2,42.85 41.45,42.85 41.95,42.35 OPTO.5 | 29.95,37.6 29.95,39.1 C11.1 | 29.95,37.6 29.95,36.6 C4.2 | 32.7,37.6 32.7,35.6 32.45,35.35 31.95,35.35 31.95,33.1 C5.2 | 29.95,37.6 32.7,37.6 | 32.7,37.6 32.95,37.85 v33.45,37.85 v41.2,37.85 41.95,37.85 42.7,37.1 C29.- 42.95,37.1 44.2,38.35 55.45,38.35 56.2,39.1 56.45,39.1 R9.2 56.7,39.1 59.2,39.1 INPUT.A12 59.45,39.1 | 63.7,19.1 62.2,19.1 59.2,22.1 40.2,22.1 38.45,20.35 R12.1
  Top 0.152: 59.45,39.1 59.45,38.85 INPUT.B1 | 59.45,39.1 59.45,40.1 59.7,40.1 INPUT.S2 59.95,40.1 63.95,40.1 INPUT.S4 | 63.95,29.1 63.95,31.35 INPUT.S3 63.95,31.6 59.95,31.6 INPUT.S1 59.7,31.6 59.45,31.6 59.45,32.35 | 46.45,32.1 46.45,30.6 46.2,30.35 45.45,30.35 PCM.16 | 46.45,32.1 45.45,32.1 PCM.19 | 59.45,32.35 59.45,32.85 INPUT.B12 | 59.45,32.35 INPUT.A1 59.2,32.35 56.45,32.35 R10.1 56.2,32.1 51.7,32.1 | 51.7,32.1 46.45,32.1 | 45.45,27.6 45.7,27.85 51.45,27.85 51.7,28.1 51.7,32.1 | 45.45,27.6 PCM.12 | 63.7,19.1 65.2,20.6 65.45,20.6 65.7,20.85 65.7,29.1 63.95,29.1 | 63.7,19.1 MIDI_IN_CONN.1 | 63.95,29.1 MIDI_OUT_CONN.1 | 5.2,18.1 1.45,18.1 1.2,18.35 1.2,20.85 2.7,20.85 5.7,23.85 5.7,26.1
  Bottom 0.152: v8.2,42.1 6.7,40.6 PWR.1 | 40.45,50.6 39.95,50.6 J3.20 | 40.45,50.6 40.95,50.6 | 40.45,50.6 J3.19 | 40.95,50.6 41.45,50.6 | 40.95,50.6 J3.18 40.95,43.1 v41.2,42.85 v41.2,37.85 | 41.45,50.6 41.95,50.6 | 41.45,50.6 J3.17 | 41.95,50.6 42.45,50.6 | 41.95,50.6 J3.16 | 43.95,51.1 J3.12 | 43.95,51.1 43.7,51.35 42.45,51.35 42.45,50.6 | 42.45,50.6 J3.15 | v47.45,51.6 J3.5 | 43.95,51.1 v44.45,51.6 | 36.45,50.6 35.95,50.6 J3.28 35.95,45.35 34.2,43.6 33.45,43.6 | 36.45,50.6 36.95,50.6 | 36.45,50.6 J3.27 | 36.95,50.6 37.45,50.6 | 36.95,50.6 J3.26 | 37.45,50.6 37.95,50.6 J3.24 | 37.45,50.6 J3.25 | J3.38 30.95,51.1 31.2,51.35 31.95,51.35 31.95,50.6 | 31.95,50.6 32.45,50.6 | 31.95,50.6 J3.36 | 32.45,50.6 32.95,50.6 | 32.45,50.6 J3.35 | 32.95,50.6 33.45,50.6 | 32.95,50.6 J3.34 | 33.45,50.6 33.95,50.6 J3.32 | 33.45,50.6 J3.33 33.45,43.6 | v33.45,37.85 33.45,43.6 | INPUT.S4 64.2,40.1 64.2,31.6 INPUT.S3
HSYNC  (via drill 0.25)
  Top 0.152: v45.45,52.6 44.45,53.6 v23.45,53.6 | v22.7,43.6 21.7,42.6 19.95,42.6 ESP32S3.33
  Bottom 0.152: v45.45,52.6 J3.9 | v23.45,53.6 22.7,52.85 v22.7,43.6
INT  (via drill 0.25)
  Top 0.152: v49.45,51.6 46.95,54.1 v25.2,54.1 | v9.2,52.1 v23.2,52.1 | v4.7,47.35 3.7,46.35 2.45,46.35 ESP32S3.5
  Bottom 0.152: v49.45,51.6 J3.1 | v23.2,52.1 v25.2,54.1 | v9.2,52.1 4.7,47.6 v4.7,47.35
IO0  (via drill 0.25)
  Top 0.152: 27.7,47.85 27.95,47.6 v28.7,47.6 | 27.7,47.85 RESET.3 | v28.7,43.1 29.45,42.35 29.7,42.35 R7.2 29.95,42.1 30.7,41.35 36.7,41.35 v36.95,41.1 | v21.2,35.35 20.45,35.35 19.95,34.85 ESP32S3.27 | 27.7,47.85 v21.7,47.85
  Bottom 0.152: v28.7,43.1 v28.7,47.6 | v21.2,35.35 21.7,35.85 v21.7,47.85 | v36.95,41.1 36.95,11.6 40.95,7.6 EXP.7
IO9  (via drill 0.25)
  Top 0.152: v12.95,28.85 10.2,31.6 6.7,31.6 6.7,33.6 ESP32S3.17
  Bottom 0.152: v12.95,28.85 14.2,27.6 14.2,5.35 19.2,0.35 40.95,0.35 40.95,4.85 43.45,7.35 EXP.8
IO38  (via drill 0.25)
  Top 0.152: v22.2,39.35 20.45,39.35 19.95,39.85 ESP32S3.31 | v23.2,34.35 v22.2,35.35 | v23.95,18.1 23.95,14.1 v31.95,14.1
  Bottom 0.152: v22.2,35.35 v22.2,39.35 | v23.2,34.35 23.95,33.6 v23.95,18.1 | v31.95,14.1 38.2,7.85 38.2,7.6 EXP.6
JOY_CLK  (via drill 0.25)
  Top 0.152: v16.2,31.1 11.95,31.1 11.95,33.6 ESP32S3.21 | v15.95,4.35 16.45,4.85 21.95,4.85 23.95,2.85 SNES.CLOCK
  Bottom 0.152: v16.2,31.1 16.2,16.6 15.95,16.35 v15.95,4.35
JOY_D0  (via drill 0.25)
  Top 0.152: v22.2,32.35 19.45,32.35 18.2,33.6 ESP32S3.26
  Bottom 0.152: v22.2,32.35 23.45,31.1 23.45,17.85 23.95,17.35 23.95,8.85 23.45,8.35 23.45,5.85 24.45,4.85 32.2,4.85 32.2,2.85 SNES.D0
JOY_LATCH  (via drill 0.25)
  Top 0.152: v16.7,34.85 16.7,33.6 ESP32S3.25
  Bottom 0.152: v16.7,34.85 16.7,16.6 16.45,16.35 16.45,12.85 22.2,7.1 22.2,2.1 23.45,0.85 28.2,0.85 28.2,2.6 SNES.LATCH
LOUT  (via drill 0.25)
  Top 0.152: 52.7,6.85 54.45,8.6 AUDIO_CONN.2 | 52.7,6.85 AUDIO_CONN.4 | v38.45,21.6 38.45,23.1 R20.1 | v42.45,16.1 43.7,17.35 C33.1 43.95,17.35 44.7,17.35 44.7,13.85 44.95,13.6 45.95,13.6 52.7,6.85
  Bottom 0.152: v38.45,21.6 39.45,20.6 39.45,17.6 40.95,16.1 v42.45,16.1
LRC  (via drill 0.25)
  Top 0.152: v46.7,29.35 45.7,29.35 45.45,29.6 PCM.15 | v45.7,8.1 43.95,6.35 27.7,6.35 26.95,7.1 26.95,9.1 11.45,9.1 v6.45,14.1 | v3.95,47.35 2.45,47.35 ESP32S3.4
  Bottom 0.152: v46.7,29.35 45.7,28.35 v45.7,8.1 | v6.45,14.1 3.95,16.6 v3.95,47.35
MIDI_IN  (via drill 0.25)
  Top 0.152: R16.1 34.2,28.1 34.2,31.1 | 34.2,31.1 20.45,31.1 19.7,31.85 16.95,31.85 15.7,33.1 15.7,33.6 ESP32S3.24 | v39.95,43.35 41.95,43.35 OPTO.6 | v38.2,32.35 36.95,31.1 34.2,31.1
  Bottom 0.152: v39.95,43.35 38.2,41.6 v38.2,32.35
MIDI_IN_SINK  (via drill 0.25)
  Top 0.152: MIDI_IN_CONN.4 50.45,14.85 54.45,18.85 MIDI_IN_CONN.2 54.45,19.1 v54.45,21.1 | v39.2,41.1 38.7,41.1 36.45,43.35 OPTO.3 | v39.95,40.35 40.45,39.85 51.7,39.85 D2.A 51.95,39.6 52.45,39.6 v53.2,38.85
  Bottom 0.152: v39.95,40.35 v39.2,41.1 | v54.45,21.1 53.2,22.35 v53.2,38.85
MIDI_IN_SOURCE  (via drill 0.25)
  Top 0.152: v52.95,41.6 51.2,41.6 50.95,41.35 46.2,41.35 43.45,44.1 40.2,44.1 38.95,45.35 32.2,45.35 31.95,45.6 R15.2 | v56.95,16.85 61.7,12.1 MIDI_IN_CONN.3 61.95,12.1 64.7,12.1 MIDI_IN_CONN.5
  Bottom 0.152: v52.95,41.6 56.95,37.6 v56.95,16.85
MIDI_OUT  (via drill 0.25)
  Top 0.152: v32.7,21.85 34.2,20.35 R18.2 | v32.2,25.1 31.2,24.1 v13.7,24.1 | v12.45,30.1 9.95,32.6 9.7,32.6 9.2,33.1 ESP32S3.19
  Bottom 0.152: v32.7,21.85 32.2,22.35 v32.2,25.1 | v13.7,24.1 12.45,25.35 v12.45,30.1
MIDI_OUT_SINK
  Top 0.152: 50.2,24.85 49.7,25.35 36.2,25.35 34.95,24.1 33.45,24.1 33.45,22.35 33.7,22.1 35.2,22.1 35.2,19.6 34.7,19.1 33.2,19.1 32.2,20.1 R18.1 | 50.2,24.85 54.45,29.1 MIDI_OUT_CONN.2 | 50.2,24.85 MIDI_OUT_CONN.4
MIDI_OUT_SOURCE
  Top 0.152: R17.2 34.45,23.1 36.2,24.85 47.7,24.85 49.95,22.6 61.2,22.6 61.7,22.1 MIDI_OUT_CONN.3 MIDI_OUT_CONN.5
N$1  (via drill 0.25)
  Top 0.152: v25.45,48.85 24.7,48.85 24.7,50.1 RESET.2 | v25.45,43.6 26.45,42.6 R1.1
  Bottom 0.152: v25.45,43.6 v25.45,48.85
N$2  (via drill 0.25)
  Top 0.152: v24.7,51.35 24.7,52.1 RESET.5 | v24.95,40.6 24.95,39.6 24.45,39.6 R6.2
  Bottom 0.152: v24.7,51.35 24.95,51.1 v24.95,40.6
N$3  (via drill 0.25)
  Top 0.152: v58.2,37.6 59.2,37.6 INPUT.B5 | v57.45,35.1 56.7,34.35 56.45,34.35 R10.2
  Bottom 0.152: v58.2,37.6 57.45,36.85 v57.45,35.1
N$7  (via drill 0.25)
  Top 0.152: v44.2,31.35 45.2,31.35 PCM.18 | v43.45,26.6 43.2,26.35 36.7,26.35 36.2,26.85 C8.1 35.2,26.85 33.95,25.6 v31.2,25.6 | v30.45,23.1 15.2,23.1 15.2,21.1 C28.+
  Bottom 0.152: v44.2,31.35 43.45,30.6 v43.45,26.6 | v30.45,23.1 31.2,23.85 v31.2,25.6
N$8  (via drill 0.25)
  Top 0.152: v40.45,13.35 40.45,11.85 R19.2 | v42.95,27.6 41.7,28.85 39.7,28.85 PCM.7
  Bottom 0.152: v40.45,13.35 42.95,15.85 v42.95,27.6
N$16  (via drill 0.25)
  Top 0.152: v41.45,30.85 39.7,30.85 PCM.4 | v42.2,24.35 43.2,23.35 43.7,23.35 C22.1
  Bottom 0.152: v41.45,30.85 42.2,30.1 v42.2,24.35
N$18  (via drill 0.25)
  Top 0.152: v43.95,29.35 41.2,32.1 39.7,32.1 PCM.2 | v44.7,24.35 45.7,23.35 C22.2
  Bottom 0.152: v43.95,29.35 44.7,28.6 v44.7,24.35
N$30  (via drill 0.25)
  Top 0.152: R15.1 29.95,45.6 30.95,44.6 36.2,44.6 OPTO.2 36.45,44.6 39.45,41.6 44.2,41.6 v44.45,41.35 | v48.7,37.1 50.95,37.1 51.7,36.35 D2.C
  Bottom 0.152: v44.45,41.35 v48.7,37.1
N$32  (via drill 0.25)
  Top 0.152: v40.45,21.6 40.45,20.35 R12.2 | v40.45,44.6 41.95,44.6 OPTO.7
  Bottom 0.152: v40.45,44.6 v40.45,21.6
N$38  (via drill 0.25)
  Top 0.152: v30.2,13.1 30.2,11.1 SERIAL.4 | v31.95,38.1 31.95,39.1 31.7,39.1 C11.2
  Bottom 0.152: v30.2,13.1 30.45,13.35 30.45,22.35 31.7,23.6 31.7,29.6 31.95,29.85 v31.95,38.1
N$42  (via drill 0.25)
  Top 0.152: v58.2,34.6 59.2,34.6 INPUT.A5 | v57.95,36.1 56.95,37.1 56.7,37.1 R9.1
  Bottom 0.152: v58.2,34.6 57.95,34.85 v57.95,36.1
OUTL  (via drill 0.25)
  Top 0.152: v41.45,24.35 40.45,23.35 R20.2 | v41.45,29.35 41.2,29.6 39.7,29.6 PCM.6
  Bottom 0.152: v41.45,29.35 v41.45,24.35
PCLK  (via drill 0.25)
  Top 0.152: v44.45,49.35 44.2,49.1 v30.95,49.1 | v15.7,22.6 v29.45,22.6 | v15.7,31.6 15.2,32.1 14.2,32.1 13.2,33.1 13.2,33.6 ESP32S3.22
  Bottom 0.152: v44.45,49.35 J3.11 | v30.95,49.1 30.45,48.6 30.45,29.6 29.45,28.6 v29.45,22.6 | v15.7,31.6 v15.7,22.6
PWM  (via drill 0.25)
  Top 0.152: v23.95,8.1 23.45,8.6 v11.45,8.6 | v9.45,39.6 8.45,40.6 3.45,40.6 2.95,41.1 2.45,41.1 ESP32S3.9
  Bottom 0.152: J3.6 46.95,49.6 43.95,46.6 43.95,32.35 45.2,31.1 45.2,10.85 42.2,7.85 42.2,7.1 40.95,5.85 23.95,5.85 v23.95,8.1 | v11.45,8.6 9.45,10.6 v9.45,39.6
R5  (via drill 0.25)
  Top 0.152: v22.2,54.6 21.45,53.85 v21.2,53.85 | v9.7,50.35 4.45,45.1 2.45,45.1 ESP32S3.6
  Bottom 0.152: J3.31 34.45,51.1 30.2,55.35 22.2,55.35 v22.2,54.6 | v21.2,53.85 20.2,52.85 20.2,52.6 19.45,51.85 9.7,51.85 v9.7,50.35
R6  (via drill 0.25)
  Top 0.152: v29.45,48.6 v34.95,48.6 | v29.2,41.1 21.95,41.1 21.7,40.85 v21.2,40.85 | v18.45,40.6 17.45,41.6 6.2,41.6 4.2,43.6 2.45,43.6 ESP32S3.7
  Bottom 0.152: v34.95,48.6 J3.30 | v29.45,48.6 29.2,48.35 v29.2,41.1 | v21.2,40.85 18.45,40.85 v18.45,40.6
R7  (via drill 0.25)
  Top 0.152: v28.2,44.1 v33.95,44.1 | v27.45,38.85 26.95,38.35 v21.2,38.35 | v18.2,38.35 15.45,41.1 6.2,41.1 4.95,42.35 2.45,42.35 ESP32S3.8
  Bottom 0.152: J3.29 35.45,45.6 v33.95,44.1 | v28.2,44.1 27.45,43.35 v27.45,38.85 | v18.2,38.35 v21.2,38.35
ROUT
  Top 0.152: 64.7,1.85 61.95,1.85 AUDIO_CONN.3 | R19.1 38.2,11.85 36.45,13.6 36.45,19.35 42.45,19.35 43.45,20.35 C32.1 43.7,20.6 44.7,21.6 54.7,21.6 58.95,17.35 65.7,17.35 65.7,8.1 64.7,7.1 64.7,1.85 | 64.7,1.85 AUDIO_CONN.5
SCL  (via drill 0.25)
  Top 0.152: v48.45,51.6 47.95,52.1 v28.45,52.1 | v26.95,34.35 26.95,33.35 26.45,33.35 R14.2 26.2,33.1 | v18.45,37.35 16.7,39.1 9.2,39.1 8.95,39.35 2.95,39.35 2.45,39.85 ESP32S3.10 | v21.45,34.35 23.7,32.1 25.2,32.1 26.2,33.1 | v29.2,9.35 33.95,9.35 35.7,7.6 EXP.5 | 26.2,33.1 v27.7,31.6
  Bottom 0.152: v48.45,51.6 J3.3 | v28.45,52.1 26.95,50.6 v26.95,34.35 | v21.45,34.35 v18.45,37.35 | v29.2,9.35 27.7,10.85 v27.7,31.6
SDA  (via drill 0.25)
  Top 0.152: v47.95,49.35 46.95,50.35 v29.2,50.35 | v28.2,46.6 27.2,45.6 R13.2 25.2,44.6 21.7,44.6 v21.2,44.1 | v15.7,38.6 2.45,38.6 ESP32S3.11
  Bottom 0.152: v47.95,49.35 J3.4 | v29.2,50.35 28.2,49.35 v28.2,46.6 | v21.2,44.1 17.2,40.1 | 17.2,40.1 v15.7,38.6 | 17.2,40.1 17.2,33.1 20.95,33.1 21.95,34.1 21.95,34.85 23.45,34.85 24.45,33.85 24.45,6.35 31.45,6.35 31.95,6.85 31.95,7.35 33.2,7.35 EXP.4
UART0_RXD  (via drill 0.25)
  Top 0.152: v15.2,14.85 18.2,11.85 27.45,11.85 27.45,11.1 SERIAL.2 | v15.2,42.1 19.2,46.1 19.7,46.1 ESP32S3.36
  Bottom 0.152: v15.2,42.1 v15.2,14.85
UART0_TXD  (via drill 0.25)
  Top 0.152: v22.95,12.35 28.7,12.35 28.7,11.1 SERIAL.3 | v21.95,11.35 17.95,11.35 v15.2,14.1 | v14.7,42.85 19.2,47.35 19.7,47.35 ESP32S3.37
  Bottom 0.152: v21.95,11.35 v22.95,12.35 | v15.2,14.1 14.7,14.6 v14.7,42.85
VNEG  (via drill 0.25)
  Top 0.152: v38.2,30.1 39.45,30.1 PCM.5 | v41.2,16.6 42.95,14.85 43.7,14.85 C23.1
  Bottom 0.152: v38.2,30.1 39.95,28.35 39.95,17.85 v41.2,16.6
VSYNC  (via drill 0.25)
  Top 0.152: v45.95,49.35 45.45,49.85 v26.45,49.85 | v25.95,44.35 25.7,44.1 21.95,44.1 21.45,43.6 19.95,43.6 ESP32S3.34
  Bottom 0.152: v45.95,49.35 J3.8 | v26.45,49.85 25.95,49.35 v25.95,44.35

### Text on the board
tNames: RESET | tulip.computer v4r7
tValues: Close
Measures: All dimensions in inches | Units: Inches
